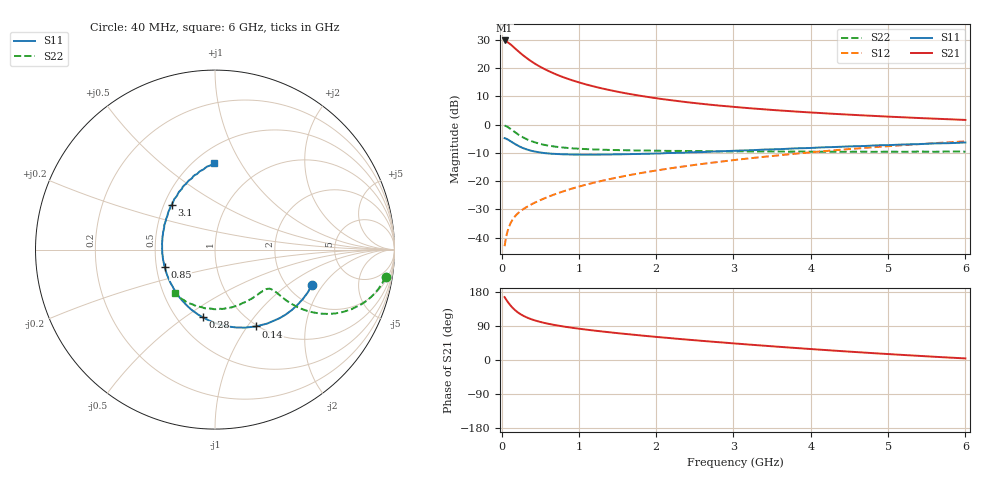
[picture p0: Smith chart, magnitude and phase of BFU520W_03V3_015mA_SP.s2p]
! Filename:  P:\Prog\Test\Noise\ATS_data\Testdata_Net\Run2\BFU520W_APM2013_06_A05_03p3V_015mA_SP_CM01_D.s2p
! Date/Time: Tue 26/Mar/2013 18:01:39
! BFU520W_APM2013_06_A05_03p3V_1to20mA_SP_CM01_Bias7_R.s2p
! MDIF S-parameter v. bias file
! BFU520W_APM2013_06_A05_03p3V_1to20mA_SP_CM01
! Date/time Tue Mar 19 16:47:37 2013
! VAR V_out= 3.3000
! VAR I_out= 15.0050
! VAR V_in= 0.8555
! VAR I_in= 0.1776
! Device data file deembeded for feedlines and parallel
! Original file: \Run2\BFU520W_APM2013_06_A05_03p3V_015mA_SP_CM01_R.s2p
! Feed-files: PR019V01_070313_Feed1.s2p, PR019V01_070313_Feed2.s2p
! Parallel-file: PR019V01_070313_Par.s2p
# MHz S MA R 50
!  Freq-MHz  S11-mag  S11-arg  S21-mag  S21-arg  S12-mag  S12-arg  S22-mag  S22-arg
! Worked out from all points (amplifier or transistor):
!   98 points, 40 MHz to 6 GHz, reference 50 ohm
!   highest |S21| = 29.7 dB at 40 MHz (marker M1)
!   |S21| within 3 dB of that: start of sweep to 182.8 MHz
!   unconditionally stable (mu >= 1): 1.056 GHz to 2.224 GHz
!   at 300 MHz: K = 0.65, MSG = 26.8 dB, |S12| = -29.6 dB
!   at 1.6 GHz: K = 1.02, MAG = 13.8 dB, |S12| = -18.2 dB
!   at 6 GHz: K = 0.85, MSG = 3.8 dB, |S12| = -6.0 dB
!   S11 on the Smith chart (normalised r, x): 40 MHz: 2.69, -1.57; 140 MHz: 0.98, -1.10; 280 MHz: 0.66, -0.59; 850 MHz: 0.55, -0.12; 3.1 GHz: 0.55, +0.31; 6 GHz: 0.62, +0.78
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40  0.5751 -19.9  30.68 166.0  0.007082 81.8  0.9624 -9.2
50  0.5695 -24.7  30.42 162.7  0.008666 80.4  0.9504 -11.3
70  0.5529 -34.0  29.13 156.5  0.0118 77.0  0.9216 -15.4
90  0.5348 -42.7  27.84 150.7  0.01465 74.0  0.8869 -19.1
120  0.5045 -54.8  25.92 143.0  0.01837 70.5  0.8307 -23.6
140  0.4848 -62.0  24.54 138.5  0.02053 68.7  0.7933 -26.0
160  0.4662 -68.8  23.16 134.4  0.02256 67.1  0.7579 -28.0
200  0.4332 -80.9  20.7 127.5  0.02606 65.3  0.6925 -31.0
240  0.4054 -91.2  18.59 121.7  0.02907 64.3  0.6383 -33.0
280  0.3832 -100.3  16.74 116.9  0.0319 64.0  0.5933 -34.2
360  0.3521 -115.0  13.86 109.6  0.03714 64.2  0.5265 -35.3
420  0.336 -123.8  12.21 105.2  0.04098 64.8  0.4909 -35.5
480  0.3246 -131.3  10.89 101.7  0.0448 65.6  0.4639 -35.4
650  0.3052 -147.5  8.322 93.8  0.05591 67.7  0.4157 -34.9
850  0.2972 -161.1  6.492 86.9  0.06945 69.4  0.3866 -35.1
1050  0.2941 -171.2  5.325 81.3  0.08346 70.4  0.3709 -36.0
1500  0.2974 171.8  3.81 70.9  0.1162 70.8  0.3538 -40.3
2050  0.3087 156.7  2.858 60.1  0.1578 69.4  0.3446 -47.7
3100  0.348 134.1  2.001 42.3  0.2437 64.0  0.3362 -66.1
4100  0.3926 117.3  1.607 27.5  0.3324 56.5  0.3305 -86.8
5200  0.4445 101.0  1.344 13.2  0.4333 46.5  0.3297 -112.2
6000  0.4823 90.4  1.208 4.2  0.5036 38.4  0.3319 -132.6
